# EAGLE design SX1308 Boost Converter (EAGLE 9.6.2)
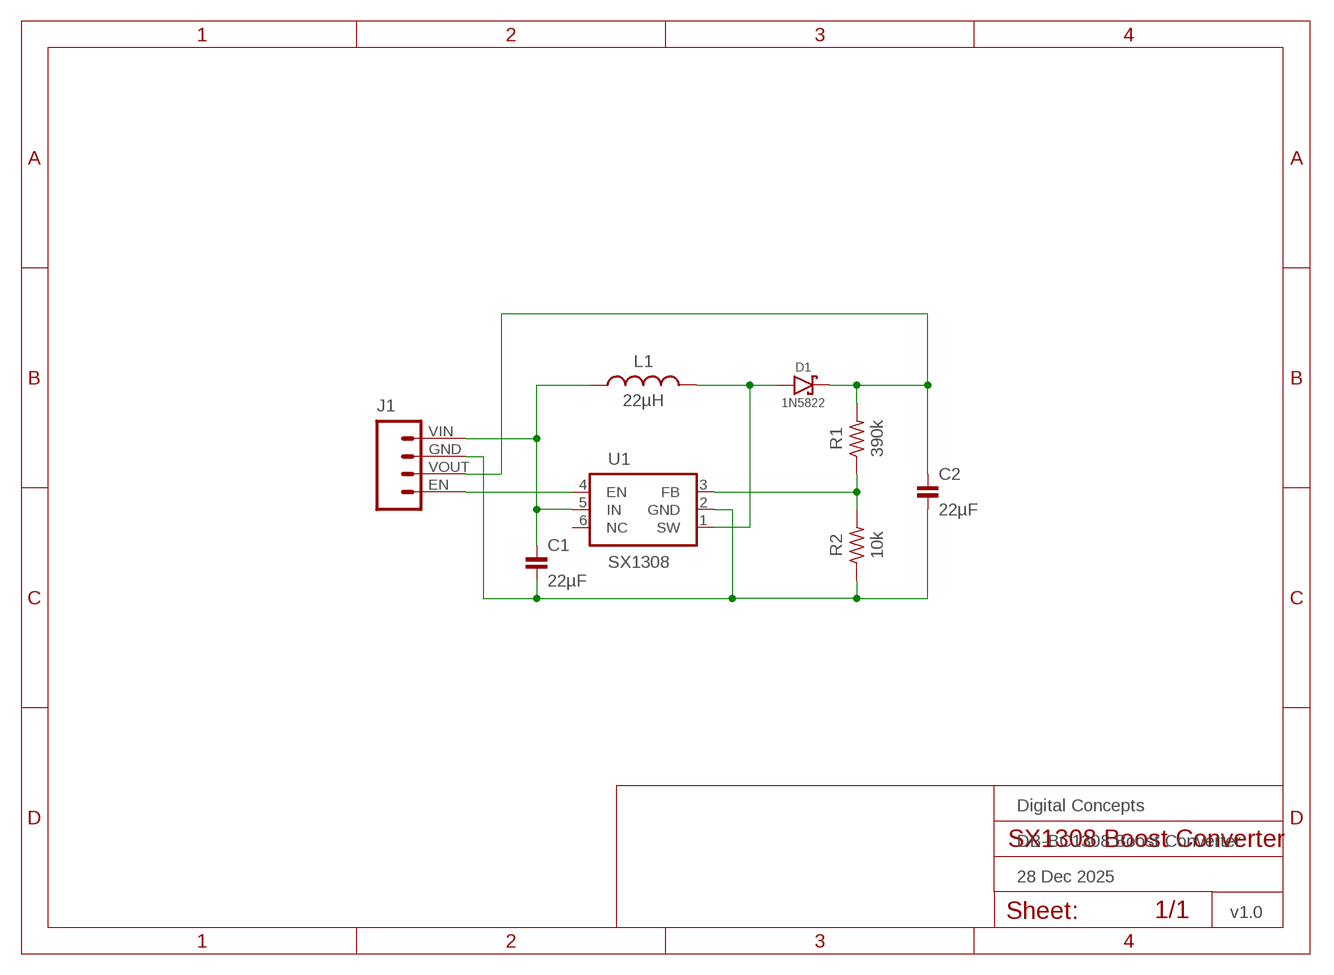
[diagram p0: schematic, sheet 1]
FRAME2 (FRAME_A5L-LOC): DATE: 28 Dec 2025; OWNER: Digital Concepts; TITLE: DB-BC1308 Boost Converter; VERSION: v1.0

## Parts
C1  22µF  CAPACITOR-0805  [C0805]
C2  22µF  CAPACITOR-0805  [C0805]
D1  1N5822  DIODE-SCHOTTKY-1N5822  [DIODE_SMB]
J1  HEADER-1X4-BOOST  [CONN_04-BOOST]
L1  22µH  INDUCTOR-CD42  [CD42]
R1  390k  RESISTOR-0603  [R0603]
R2  10k  RESISTOR-0603  [R0603]
U1  SX1308  [SOT-23-6]

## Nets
28V: C2.1 D1.C J1.VOUT R1.2
EN: J1.EN U1.4(EN)
GND: C1.2 C2.2 J1.GND R2.1 U1.2(GND)
N$1: D1.A L1.P$1 U1.1(SW)
N$3: R1.1 R2.2 U1.3(FB)
VIN: C1.1 J1.VIN L1.P$2 U1.5(IN)
Unconnected: U1.6(NC)

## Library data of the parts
C1 C2 = digitalconcepts:CAPACITOR-0805: 0805 Capacitor
D1 = digitalconcepts:DIODE-SCHOTTKY-1N5822: 1N5822 Schottky Diode SMB
J1 = digitalconcepts:HEADER-1X4-BOOST: Boost Converter Module 4-Pin Header
L1 = digitalconcepts:INDUCTOR-CD42: CD42 Inductor
R1 R2 = digitalconcepts:RESISTOR-0603: Resistor
U1 = digitalconcepts:SX1308: MT3608 DC-DC Step-Up Voltage Converter

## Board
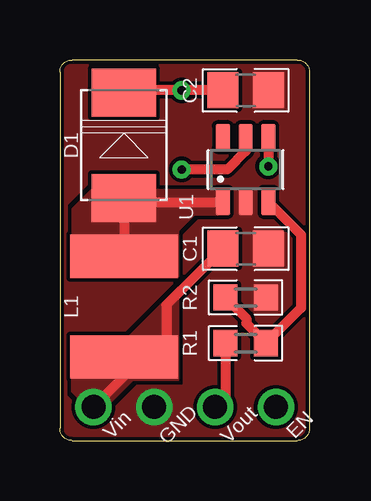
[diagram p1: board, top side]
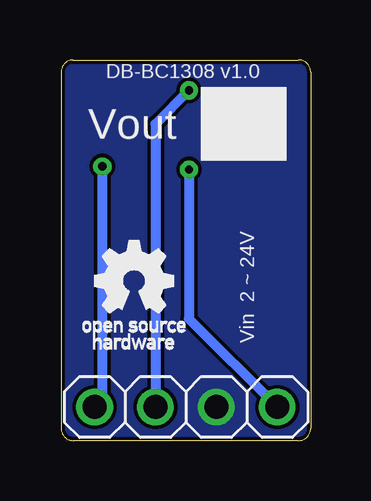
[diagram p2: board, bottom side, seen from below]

Size 10.41 x 15.88 mm. Coordinates in mm from the lower left corner, seen from the top.
Outline: 9.91,15.88 arc-90 10.41,15.37 10.41,0.51 arc-90 9.91,0 0.51,0 arc-90 0,0.51 0,15.37 arc-90 0.51,15.88 9.91,15.88
Copper layers (1*16): Top 0.035mm / dielectric 1.5mm / Bottom 0.035mm
Design rules "default *": minimum track width 6mil, minimum drill 0.15mm, track to track 6mil, track to pad 6mil, pad to pad 6mil, via to via 6mil, smd to smd 6mil, copper to edge 6mil, drill to drill 6mil, minimum pad ring 10mil, minimum via ring 8mil, stop-mask expansion 4mil, vias tented up to drill 0mil, thermal gap 0mil

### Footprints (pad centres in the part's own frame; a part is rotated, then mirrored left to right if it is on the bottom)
C0805 = smd 1.3 x 1.5: 1 -0.95,0; 2 0.95,0
DIODE_SMB = smd 2 x 2.7: A 2.2,0; C -2.2,0
CONN_04-BOOST = drill 1 pad 1.524: EN 0,0; GND 5.08,0; VIN 7.62,0; VOUT 2.54,0
CD42 = smd 4.5 x 1.8: P$1 0,2.1; P$2 0,-2.1
R0603 = smd 1 x 1.1: 1 -0.85,0; 2 0.85,0
SOT-23-6 = smd 1.1 x 0.6: 1 -1.35,0.95; 2 -1.35,0; 3 -1.35,-0.95; 4 1.35,-0.95; 5 1.35,0; 6 1.35,0.95

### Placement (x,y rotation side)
C1  7.75,8 0 top
C2  7.75,14.61 0 top
D1  2.67,12.32 270 top
J1  9.02,1.4 0 bottom
L1  2.67,5.59 0 top
R1  7.75,4.06 180 top
R2  7.75,5.97 180 top
U1  7.75,11.3 90 top

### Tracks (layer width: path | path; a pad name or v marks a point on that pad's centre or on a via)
28V  (via drill 0.35)
  Top 0.406: R1.2 6.9,1.82 J1.VOUT | D1.C 3.01,14.61 v5.08,14.61 C2.1
  Bottom 0.406: v5.08,14.61 6.48,13.21 J1.VOUT
EN  (via drill 0.35)
  Top 0.406: U1.4 v8.7,11.43
  Bottom 0.406: v8.7,11.43 8.7,1.72 J1.EN
GND
  pour Top (rank 5): -0.51,16.38 10.92,16.38 10.92,-0.51 -0.51,-0.51
  pour Bottom: -0.25,16.13 10.67,16.13 10.67,-0.25 -0.25,-0.25
N$1
  Top 0.406: L1.P$1 D1.A 2.75,9.95 U1.1
  pour Top (no thermals): 6.6,9.42 6.6,10.44 1.3,10.44 0.51,9.65 0.51,6.86 4.95,6.86 4.95,8.76 5.61,9.42
N$3
  Top 0.406: R2.2 7.77,5.09 7.77,4.89 R1.1 10.06,5.53 10.06,8.59 U1.3
VIN  (via drill 0.35)
  Top 0.406: J1.VIN 2.67,2.67 L1.P$2 3.94,3.49 4.45,4 4.45,5.65 C1.1 | U1.5 7.75,12.06 6.99,11.3 v5.08,11.3
  Bottom 0.406: v5.08,11.3 5.08,5.08 J1.VIN
  pour Top (no thermals): 0.48,2.06 1.27,1.27 1.78,1.27 3.05,2.54 4.95,2.54 4.95,6.4 2.87,4.32 0.48,4.32

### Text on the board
bPlace: DB-BC1308 v1.0 | Vout | Vin 2 ~ 24V
tNames: Vin | GND | Vout | EN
